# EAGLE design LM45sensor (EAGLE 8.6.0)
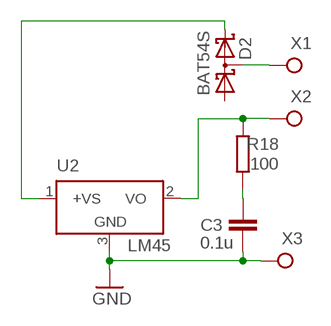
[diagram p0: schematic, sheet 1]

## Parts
C3  0.1u  C-EUC0805  [C0805]
D2  BAT54S  [SOT23]
R18  100  R-EU_R0805  [R0805]
U2  LM45  LM50  [SOT23]
X1  TPPAD1-13  [P1-13]
X2  TPPAD1-13  [P1-13]
X3  TPPAD1-13  [P1-13]

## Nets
GND: C3.2 U2.3(GND) X3.TP
N$1: D2.3(C1A2) X1.TP
N$2: D2.2(C2) U2.1(+VS)
N$3: R18.2 U2.2(VO) X2.TP
N$5: C3.1 R18.1
Unconnected: D2.1(A1)

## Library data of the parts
C3 = rcl:C-EU: CAPACITOR, European symbol
D2 = diode:BAT54S: Schottky Diodes Pin connection corrected 2011-05-04 Source: Fairchild .. BAT54.pdf
R18 = rcl:R-EU_: RESISTOR, European symbol
U2 = linear:LM50: SOT-23 Single-Supply Centigrade Temperature Sensor Vout = (10mV/°C x Temp °C) +5mmmV Source: http://cache.national.com/ds/LM/LM50.pdf
X1-X3 = testpad:TP: Test pad

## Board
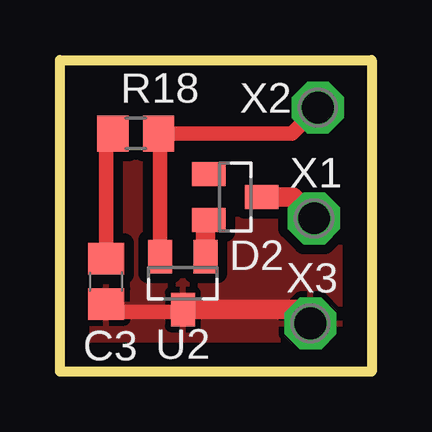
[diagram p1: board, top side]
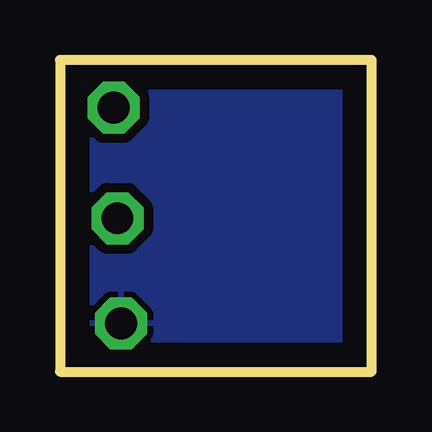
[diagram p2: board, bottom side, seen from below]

Size 13 x 13 mm. Coordinates in mm from the lower left corner, seen from the top.
Outline: 0,0 0,13 13,13 13,0 0,0
Copper layers (1*16): Top 0.035mm / dielectric 1.5mm / Bottom 0.035mm
Design rules "default": minimum track width 10mil, minimum drill 24mil, track to track 8mil, track to pad 8mil, pad to pad 8mil, via to via 8mil, smd to smd 8mil, copper to edge 40mil, drill to drill 8mil, minimum pad ring 10mil, minimum via ring 8mil, stop-mask expansion 4mil, vias tented up to drill 0mil, thermal gap 10mil

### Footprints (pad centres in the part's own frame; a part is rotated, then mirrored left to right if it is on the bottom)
C0805 = smd 1.3 x 1.5: 1 -0.95,0; 2 0.95,0
SOT23 = smd 1 x 1.4: 1 -0.95,-1.1; 2 0.95,-1.1; 3 0,1.1
R0805 = smd 1.3 x 1.5: 1 -0.95,0; 2 0.95,0
P1-13 = drill 1.321 pad 2.159 octagon: TP 0,0

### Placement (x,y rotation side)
C3  1.93,3.76 270 top
D2  7.31,7.28 270 top
R18  3.16,9.93 0 top
U2  5.13,3.69 180 top
X1  10.6,6.39 0 top
X2  10.76,11.01 0 top
X3  10.45,2.01 0 top

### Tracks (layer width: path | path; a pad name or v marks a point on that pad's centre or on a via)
GND
  Top 0.61: C3.2 2.19,2.81 2.5,2.5 5.04,2.5 U2.3
  Top 0.813: U2.3 9.87,2.59 X3.TP
  pour Top (isolate 0.406): 0.5,12.75 12.5,12.75 12.5,0.25 0.5,0.25
  pour Bottom (isolate 0.4): 0.5,12.5 12.25,12.5 12.25,0.5 0.5,0.5
N$1
  Top 0.813: D2.3 9.71,7.28 X1.TP
N$2
  Top 0.813: U2.1 6.08,6.2 D2.2
N$3
  Top 0.61: U2.2 4.18,9.86 R18.2 9.68,9.93 X2.TP
N$5
  Top 0.61: C3.1 1.93,9.65 R18.1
